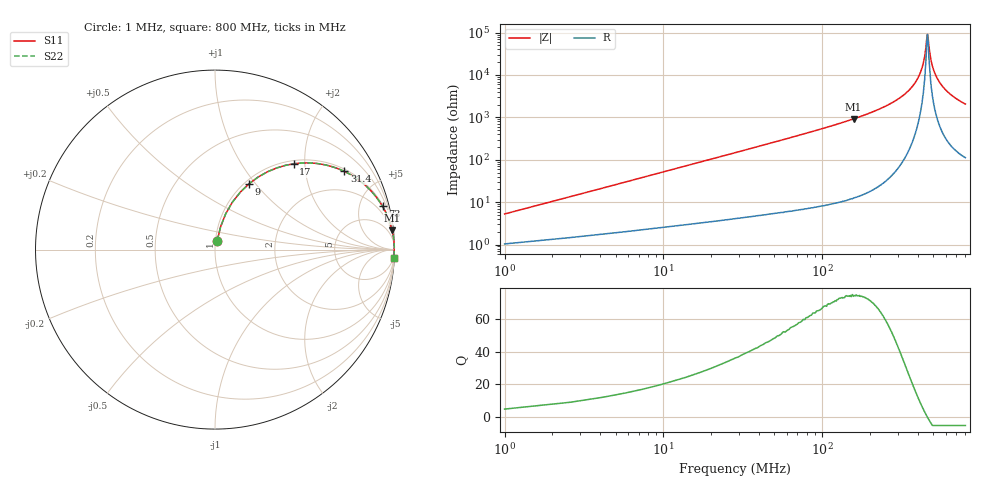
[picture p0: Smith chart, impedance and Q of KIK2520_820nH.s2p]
!version-2
!date-01.2022
!Series
# MHz S RI R 50
!Freq ReS11 ImS11 ReS21 ImS21 ReS12 ImS12 ReS22 ImS22
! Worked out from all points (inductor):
!   501 points, 1 MHz to 800 MHz, reference 50 ohm
!   read as one part in series: L = 820 nH near 4.2 MHz
!   highest Q = 74.2 at 158 MHz (marker M1), where L = 928 nH
!   self-resonance near 460 MHz
!   S11 on the Smith chart (normalised r, x): 1 MHz: 1.02, +0.10; 9 MHz: 1.05, +0.93; 17 MHz: 1.06, +1.75; 31.4 MHz: 1.09, +3.25; 73 MHz: 1.13, +7.72; 800 MHz: 3, -41
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1  0.0128 0.0503  0.9872 -0.0503  0.9872 -0.0503  0.0128 0.0503
5.8  0.0972 0.2645  0.9028 -0.2645  0.9028 -0.2645  0.0972 0.2645
9  0.1898 0.3669  0.8102 -0.3669  0.8102 -0.3669  0.1898 0.3669
17  0.4374 0.4781  0.5626 -0.4781  0.5626 -0.4781  0.4374 0.4781
31.4  0.7204 0.4359  0.2796 -0.4359  0.2796 -0.4359  0.7204 0.4359
47.4  0.8538 0.3428  0.1462 -0.3428  0.1462 -0.3428  0.8538 0.3428
73  0.9334 0.2408  0.0666 -0.2408  0.0666 -0.2408  0.9334 0.2408
135  0.9814 0.1283  0.0186 -0.1283  0.0186 -0.1283  0.9814 0.1283
158  0.9869 0.107  0.0131 -0.107  0.0131 -0.107  0.9869 0.107
268  0.9968 0.0477  0.00317 -0.0477  0.00317 -0.0477  0.9968 0.0477
347  0.9985 0.0244  0.00148 -0.0244  0.00148 -0.0244  0.9985 0.0244
401  0.9989 0.0118  0.0011 -0.0118  0.0011 -0.0118  0.9989 0.0118
435  0.9989 0.00507  0.00106 -0.00507  0.00106 -0.00507  0.9989 0.00507
462  0.9989 -2.83e-05  0.00111 2.83e-05  0.00111 2.83e-05  0.9989 -2.83e-05
467  0.9989 -0.000895  0.00112 0.000895  0.00112 0.000895  0.9989 -0.000895
479  0.9988 -0.00316  0.00117 0.00316  0.00117 0.00316  0.9988 -0.00316
487  0.9988 -0.00455  0.0012 0.00455  0.0012 0.00455  0.9988 -0.00455
511  0.9987 -0.0086  0.00133 0.0086  0.00133 0.0086  0.9987 -0.0086
534  0.9985 -0.0122  0.00149 0.0122  0.00149 0.0122  0.9985 -0.0122
591  0.998 -0.0209  0.002 0.0209  0.002 0.0209  0.998 -0.0209
667  0.9971 -0.0314  0.0029 0.0314  0.0029 0.0314  0.9971 -0.0314
800  0.995 -0.0482  0.00497 0.0482  0.00497 0.0482  0.995 -0.0482
